(* Logix 5000 AddOnInstructionDefinition export AMCI_MA_SV_Circular_Follower_CIPSync; software revision 20.05 *)

TYPE AMCI_Motion_Axis_Output_Data :
STRUCT
   Control_Word_0 : INT;
   Control_Word_1 : INT;
   Position_or_Distance : DINT;
   Programmed_Speed : DINT;
   Acceleration : INT;
   Deceleration : INT;
   Output_Word_8 : INT;
   Output_Word_9 : INT;
END_STRUCT
END_TYPE

TYPE AMCI_Motion_Axis_Input_Data :
STRUCT
   Moving_CW : BOOL;
   Moving_CCW : BOOL;
   In_Hold_State : BOOL;
   Stopped : BOOL;
   At_Home : BOOL;
   Accelerating : BOOL;
   Decelerating : BOOL;
   Move_Complete : BOOL;
   Status_Word_0_Bit_8 : BOOL;
   Status_Word_0_Bit_9 : BOOL;
   Position_Invalid : BOOL;
   Input_Error : BOOL;
   Command_Error : BOOL;
   Configuration_Error : BOOL;
   Module_OK : BOOL;
   Mode_Flag : BOOL;
   IN1_Active : BOOL;
   IN2_Active : BOOL;
   IN3_Active : BOOL;
   IN4_Active : BOOL;
   Status_Word_1_Bit_4 : BOOL;
   Status_Word_1_Bit_5 : BOOL;
   Connection_Was_Lost : BOOL;
   Driver_Fault : BOOL;
   Status_Word_1_Bit_8 : BOOL;
   Invalid_Jog_Change : BOOL;
   Status_Word_1_Bit_10 : BOOL;
   Heartbeat_Bit : BOOL;
   Status_Word_1_Bit_12 : BOOL;
   Status_Word_1_Bit_13 : BOOL;
   Stall_Detected : BOOL;
   Drive_Is_Enabled : BOOL;
   Motor_Position : DINT;
   Encoder_Position : DINT;
   Trapped_Encoder_Position : DINT;
   Input_Word_8 : INT;
   Input_Word_9 : INT;
END_STRUCT
END_TYPE

ADD_ON_INSTRUCTION AMCI_MA_SV_Circular_Follower_CIPSync   (* revision 1.0, vendor AMCI, ExecuteEnableInFalse *)
// Only for SVXXXE2 motion devices.
// Revision note:
// 8/8/24.  Added CIPSync functionality to a previously existing AOI.  The abiltiy to change the maximum move torque is no longer available because the time value uses the same output words as the torque value.
// Help:
// MOTION AXIS SV CIRCULAR FOLLOWER
// These AOIs will only work with the SD and SMD motion devices.  The SV motion devices have their own follower AOIs.
// AXIS INPUT DATA:  Input data from AMCI motion device.   Uses the AMCI_Motion_Axis_Input_Data User Defined Data Type.
// AXIS OUTPUT DATA; Output data from the AOI to the AMCI motion device.   Uses the AMCI_Motion_Axis_Output_Data User Defined Data Type.
// FOLLOWER POSITION: REAL DATA TYPE position directly from the motion axis.
// FOLLOWER VELOCITY: REAL DATA TYPE velocity directly from the motion axis.
// FOLLOWER ACCELERATION: REAL DATA TYPE acceleration directly from the motion axis.
// RAMP ACCELERATION: An actual value or INT value used to transition from no motion to motion.   Once
//                                          motion is occurring, the follower acceleration will be used.  Range of 0 to 15,999.
// DECELERATION: An actual value or INT value used to transition from motion to no motion.   Range of 0 to
//                              15,999.
// CONVERSION CONSTANT: Converts revolutions and revolutions / sec  from the motion axis to the step and
//                                               steps / sec used by the motion axis.
// POSITION UNWIND: Must be set to the Unwind Value of the motion axis and defines the point at which the
//                                    position data will transition from its maximum to its minimum value.    The Position
//                                    Unwind Value MUST BE IN THE RANGE OF 21 TO 65535.
// EN (Enable) Set when rung is true, Reset when rung is false
// DN (Done) Set when command is sent to the motion device.  Reset when the rung is false.
// ER (Error) Set when a command or input error failed to clear.  Reset when the rung is false.
// IP (In Process) Set when motion is occurring.   Reset when the rung goes false.
VAR_IN_OUT
   Axis_Input_Data : AMCI_Motion_Axis_Input_Data; {required}
   Axis_Output_Data : AMCI_Motion_Axis_Output_Data; {required}
END_VAR
VAR_INPUT
   current_system_time : DINT; {required}
   Master_Axis_Position : REAL; {required}
   Master_Axis_Velocity : REAL; {required}
   Master_Acceleration : REAL; {required}
   Ramp_Acceleration : INT; {required}
   Deceleration : INT; {required}
   Conversion_Constant : REAL; {required}
   Position_Unwind : DINT; {required}
END_VAR
VAR_OUTPUT
   EN : BOOL; {visible}
   ER : BOOL; {visible}
   DN : BOOL; {access Read Only, visible}
   IP : BOOL; {access Read Only, visible}
END_VAR
VAR
   command_data_block : INT[10];
        [0]   // Command Bits MSW
        [1]   // Command Bits LSW
        [2]   // Upper Target Position
        [3]   // Lower Target Position
        [4]   // Upper Programmed Speed
        [5]   // Lower Programmed Speed
        [8]   // Unwind value when stopped, Maximum Move Torque when motion occurring
   axis_follower_position : DINT;
   axis_follower_velocity : DINT;
   axis_follower_acceleration : DINT; {access None}
END_VAR

ROUTINE EnableInFalse   (* ladder *)
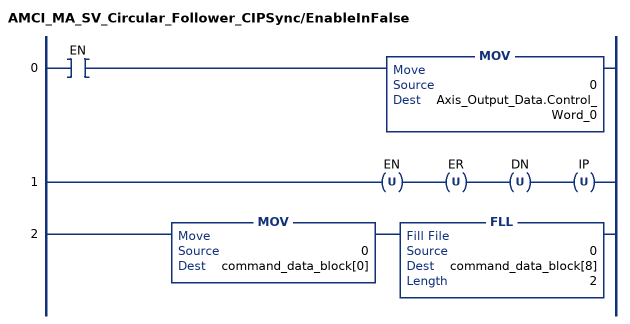
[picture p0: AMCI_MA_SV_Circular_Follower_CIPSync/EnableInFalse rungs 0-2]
   0: XIC(EN)MOV(0,Axis_Output_Data.Control_Word_0);
   1: OTU(EN)OTU(ER)OTU(DN)OTU(IP);
   2: MOV(0,command_data_block[0])FLL(0,command_data_block[8],2);
END_ROUTINE

ROUTINE Logic   (* ladder *)
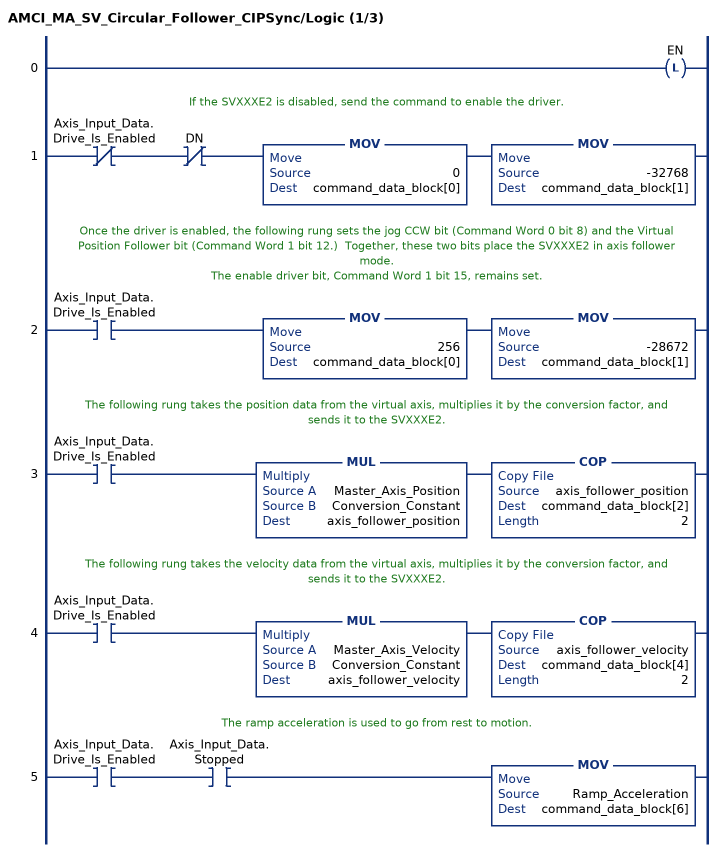
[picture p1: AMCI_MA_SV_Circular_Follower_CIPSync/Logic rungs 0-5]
   0: OTL(EN);
   // If the SVXXXE2 is disabled, send the command to enable the driver.
   1: XIO(Axis_Input_Data.Drive_Is_Enabled)XIO(DN)MOV(0,command_data_block[0])MOV(-32768,command_data_block[1]);
   // Once the driver is enabled, the following rung sets the jog CCW bit (Command Word 0 bit 8) and the Virtual Position Follower bit (Command Word 1 bit 12.)  Together, these two bits place the SVXXXE2 in axis follower mode.
   // The enable driver bit, Command Word 1 bit 15, remains set.
   2: XIC(Axis_Input_Data.Drive_Is_Enabled)MOV(256,command_data_block[0])MOV(-28672,command_data_block[1]);
   // The following rung takes the position data from the virtual axis, multiplies it by the conversion factor, and sends it to the SVXXXE2.
   3: XIC(Axis_Input_Data.Drive_Is_Enabled)MUL(Master_Axis_Position,Conversion_Constant,axis_follower_position)COP(axis_follower_position,command_data_block[2],2);
   // The following rung takes the velocity data from the virtual axis, multiplies it by the conversion factor, and sends it to the SVXXXE2.
   4: XIC(Axis_Input_Data.Drive_Is_Enabled)MUL(Master_Axis_Velocity,Conversion_Constant,axis_follower_velocity)COP(axis_follower_velocity,command_data_block[4],2);
   // The ramp acceleration is used to go from rest to motion.
   5: XIC(Axis_Input_Data.Drive_Is_Enabled)XIC(Axis_Input_Data.Stopped)MOV(Ramp_Acceleration,command_data_block[6]);
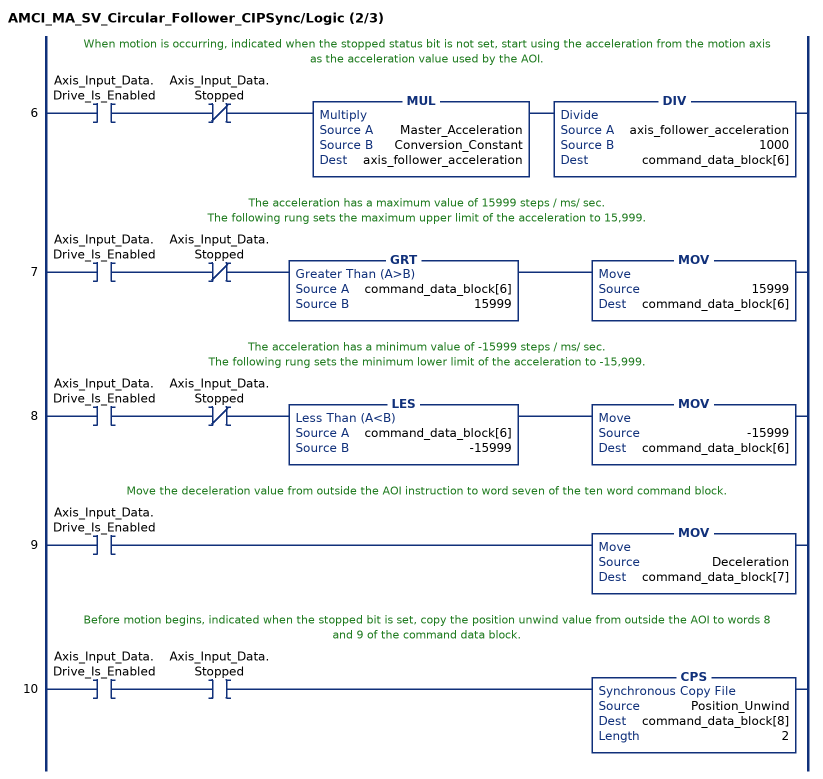
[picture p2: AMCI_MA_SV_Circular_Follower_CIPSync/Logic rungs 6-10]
   // When motion is occurring, indicated when the stopped status bit is not set, start using the acceleration from the motion axis as the acceleration value used by the AOI.
   6: XIC(Axis_Input_Data.Drive_Is_Enabled)XIO(Axis_Input_Data.Stopped)MUL(Master_Acceleration,Conversion_Constant,axis_follower_acceleration)DIV(axis_follower_acceleration,1000,command_data_block[6]);
   // The acceleration has a maximum value of 15999 steps / ms/ sec.
   // The following rung sets the maximum upper limit of the acceleration to 15,999.
   7: XIC(Axis_Input_Data.Drive_Is_Enabled)XIO(Axis_Input_Data.Stopped)GRT(command_data_block[6],15999)MOV(15999,command_data_block[6]);
   // The acceleration has a minimum value of -15999 steps / ms/ sec.
   // The following rung sets the minimum lower limit of the acceleration to -15,999.
   8: XIC(Axis_Input_Data.Drive_Is_Enabled)XIO(Axis_Input_Data.Stopped)LES(command_data_block[6],-15999)MOV(-15999,command_data_block[6]);
   // Move the deceleration value from outside the AOI instruction to word seven of the ten word command block.
   9: XIC(Axis_Input_Data.Drive_Is_Enabled)MOV(Deceleration,command_data_block[7]);
   // Before motion begins, indicated when the stopped bit is set, copy the position unwind value from outside the AOI to words 8 and 9 of the command data block.
   10: XIC(Axis_Input_Data.Drive_Is_Enabled)XIC(Axis_Input_Data.Stopped)CPS(Position_Unwind,command_data_block[8],2);
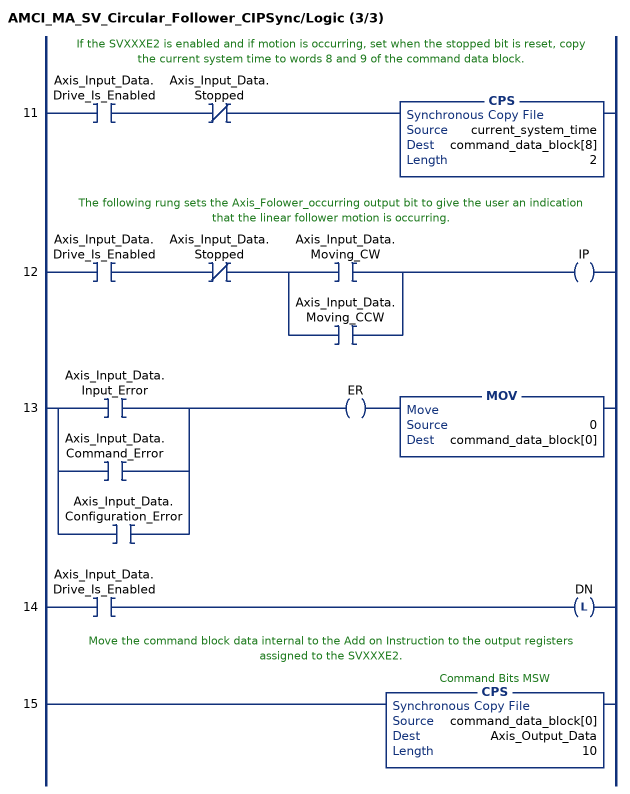
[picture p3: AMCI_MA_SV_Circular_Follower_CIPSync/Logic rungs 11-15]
   // If the SVXXXE2 is enabled and if motion is occurring, set when the stopped bit is reset, copy the current system time to words 8 and 9 of the command data block.
   11: XIC(Axis_Input_Data.Drive_Is_Enabled)XIO(Axis_Input_Data.Stopped)CPS(current_system_time,command_data_block[8],2);
   // The following rung sets the Axis_Folower_occurring output bit to give the user an indication that the linear follower motion is occurring.
   12: XIC(Axis_Input_Data.Drive_Is_Enabled)XIO(Axis_Input_Data.Stopped)[XIC(Axis_Input_Data.Moving_CW) ,XIC(Axis_Input_Data.Moving_CCW) ]OTE(IP);
   13: [XIC(Axis_Input_Data.Input_Error) ,XIC(Axis_Input_Data.Command_Error) ,XIC(Axis_Input_Data.Configuration_Error) ]OTE(ER)MOV(0,command_data_block[0]);
   14: XIC(Axis_Input_Data.Drive_Is_Enabled)OTL(DN);
   // Move the command block data internal to the Add on Instruction to the output registers assigned to the SVXXXE2.
   15: CPS(command_data_block[0],Axis_Output_Data,10);
END_ROUTINE
END_ADD_ON_INSTRUCTION
